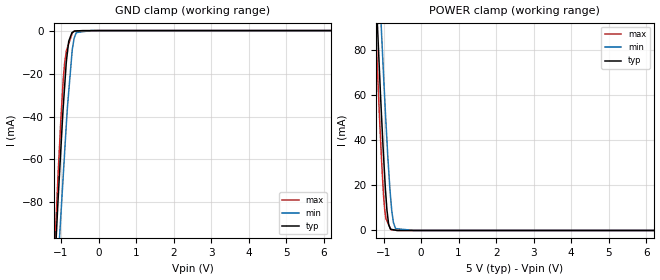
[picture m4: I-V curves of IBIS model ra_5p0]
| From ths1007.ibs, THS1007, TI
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|   ra_5p0 Model
[Model]   ra_5p0
Model_type   Input
Vinl = 0.6
Vinh = 2.6
|   typ   min   max
|   (nom PVT)   (fast PVT)   (slow PVT)
C_comp   9.560e-13   9.523e-13   9.597e-13
| Where nom  PVT is Nominal Process, 5V, 27C
| Fast PVT is Strong Process,  5.25V, -40C
| Slow PVT is Weak Process,   4.75V, 125C
[Voltage Range]   5   4.75   5.25
|Ambient Temperature   25   85   -40
|Junction Temperature
[Temperature Range]   27   125   -40
[Power Clamp Reference]   5   4.75   5.25
[GND Clamp Reference]   0   0   0
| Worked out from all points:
|   GND clamp passes 1 mA (typ) near -0.71 V on its own axis
|   POWER clamp passes 1 mA (typ) near -0.83 V on its own axis
[GND Clamp]
|   Voltage   I(typ)   I(min)   I(max)
-5V       -1.711A    -1.633A    -1.808A
-1.306V   -159mA     -183.6mA   -155.6mA
-1.088V   -81.72mA   -111.6mA   -70.6mA
-1.031V   -63.44mA   -93.66mA   -50.5mA
-934.5mV  -33.8mA    -65.6mA    -21.24mA
-855mV    -13.85mA   -42.43mA   -9.274mA
-795mV    -4.987mA   -28.46mA   -6.115mA
-703mV    -917.8uA   -9.275mA   -1.272mA
-640mV    -213.3uA   -3.007mA   -237.7uA
-593.8mV  -169.5uA   -912.7uA   -220.5uA
-190mV    0A         -23.35nA   -70.56uA
10V       0A         0A         0A
[POWER Clamp]
|   Voltage   I(typ)   I(min)   I(max)
-5V       1.711A     1.714A     1.72A
-1.306V   144.9mA    181.1mA    127mA
-1.113V   72.14mA    109.1mA    52.07mA
-1.054V   50.94mA    87.81mA    31.8mA
-966mV    22.96mA    57.47mA    8.774mA
-910mV    9.161mA    39.94mA    4.269mA
-860mV    2.43mA     25.95mA    2.444mA
-803.3mV  525.6uA    13.03mA    372.2uA
-736.2mV  316.1uA    3.495mA    231.3uA
-679.3mV  137.9uA    817.9uA    111.4uA
-190mV    0A         0A         8.884uA
10V       0A         0A         0A
